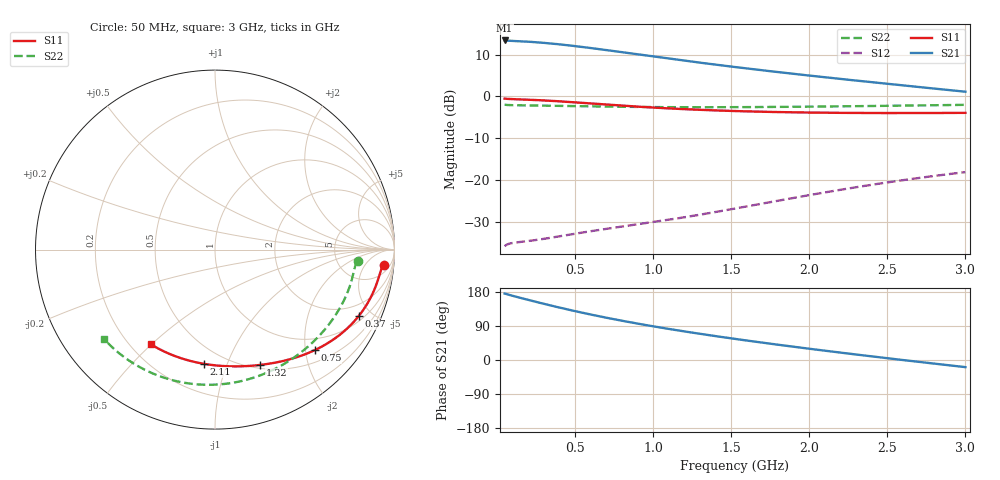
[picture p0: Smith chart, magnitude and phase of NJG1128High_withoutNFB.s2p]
! NJG1128 High Gain mode S-parameter
# hz S ma R 50	S	ma	R	50
! 2 Port Network Data from SP1.SP block	Port	Network	Data	from	SP1.SP	block
! freq  magS11  angS11  magS21  angS21  magS12  angS12  magS22  angS22  magS11	angS11	magS21	angS21	magS12	angS12	magS22	angS22
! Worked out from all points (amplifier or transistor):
!   591 points, 50 MHz to 3 GHz, reference 50 ohm
!   highest |S21| = 13.4 dB at 50 MHz (marker M1)
!   |S21| within 3 dB of that: start of sweep to 841 MHz
!   unconditionally stable (mu >= 1): 83.52 MHz to 2.291 GHz
!   at 540 MHz: K = 1.18, MAG = 19.6 dB, |S12| = -32.5 dB
!   at 1.525 GHz: K = 1.35, MAG = 13.4 dB, |S12| = -26.7 dB
!   at 3 GHz: K = 0.76, MSG = 9.6 dB, |S12| = -18.1 dB
!   lowest NFmin = 0.65 dB at 300 MHz
!   S11 on the Smith chart (normalised r, x): 50 MHz: 10, -15; 370 MHz: 1.25, -4.18; 750 MHz: 0.74, -2.19; 1.32 GHz: 0.54, -1.32; 2.11 GHz: 0.39, -0.83; 3 GHz: 0.28, -0.50
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5e7  0.9427 -5.2  4.657 175.5  0.01636 30.5  0.7969 -4.7
1.4e8  0.9238 -10.4  4.565 165.2  0.01829 20.3  0.7844 -8.3
2.2e8  0.9119 -15.5  4.476 156.6  0.01904 22.2  0.781 -12.2
2.95e8  0.8981 -20.2  4.369 148.9  0.01993 25.2  0.7777 -15.9
3.7e8  0.882 -24.9  4.242 141.4  0.02099 28.2  0.774 -19.6
4.55e8  0.8617 -29.9  4.081 133.2  0.02231 31.3  0.7695 -23.8
5.45e8  0.8392 -34.9  3.899 125.0  0.02376 34.0  0.7647 -28.2
6.45e8  0.8142 -40.1  3.692 116.3  0.0254 36.7  0.7596 -33.0
7.5e8  0.789 -45.2  3.477 107.6  0.02715 39.2  0.7549 -37.9
8.9e8  0.7585 -51.6  3.203 96.9  0.02959 42.3  0.75 -44.4
1.035e9  0.7312 -57.7  2.943 86.5  0.0324 45.4  0.7464 -51.0
1.175e9  0.7091 -63.2  2.716 77.1  0.03555 48.2  0.7445 -57.3
1.32e9  0.6903 -68.6  2.505 67.9  0.0394 50.6  0.744 -63.9
1.42e9  0.6795 -72.2  2.372 61.9  0.04244 51.8  0.7443 -68.4
1.525e9  0.6698 -75.9  2.244 55.7  0.046 52.9  0.7453 -73.2
1.76e9  0.6534 -83.9  1.993 42.5  0.05528 53.7  0.7493 -83.9
2.02e9  0.6421 -92.6  1.759 28.7  0.06753 52.4  0.7561 -95.8
2.11e9  0.6394 -95.5  1.687 24.1  0.07219 51.5  0.759 -100.0
2.31e9  0.6355 -102.0  1.541 14.0  0.08318 48.7  0.766 -109.2
2.51e9  0.6338 -108.4  1.41 4.2  0.09489 45.0  0.7737 -118.5
2.755e9  0.6344 -116.2  1.267 -7.4  0.1099 39.4  0.7839 -129.8
3e9  0.6374 -124.0  1.139 -18.8  0.1251 32.9  0.7943 -141.2
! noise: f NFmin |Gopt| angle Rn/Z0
5e+07  0.9186  0.831  7.566  1.126
3.75e+08  0.6501  0.6638  21.44  0.3463
7.05e+08  0.6855  0.6386  37.42  0.3162
1.03e+09  0.7402  0.6109  53.48  0.2844
1.36e+09  0.8077  0.5799  69.62  0.2471
1.685e+09  0.8819  0.5487  85.2  0.2085
2.015e+09  0.9628  0.5185  100.6  0.1709
2.34e+09  1.048  0.4916  115.1  0.1386
2.67e+09  1.14  0.4686  129.3  0.1125
3e+09  1.242  0.4516  142.6  0.094
